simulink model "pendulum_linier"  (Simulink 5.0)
settings: Solver=ode45  StartTime=0.0  StopTime=25  RelTol=1e-6
libraries: simulink x1

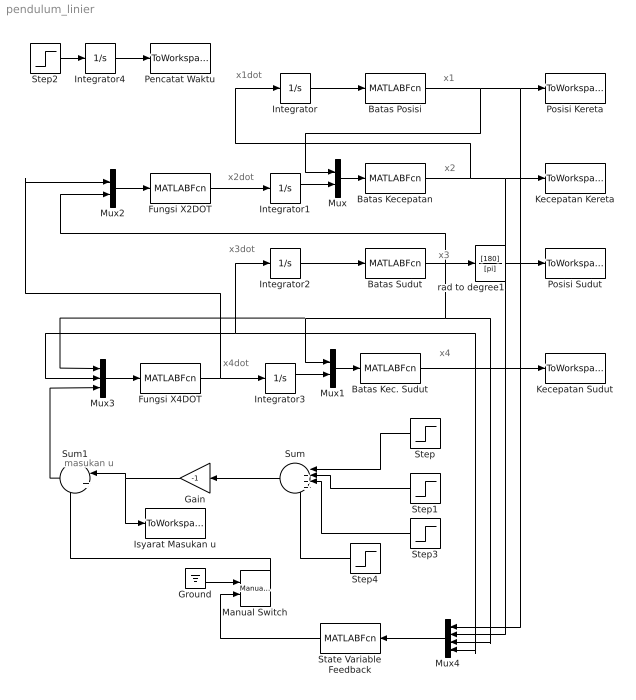
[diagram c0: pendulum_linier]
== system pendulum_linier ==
  note: x1
  note: x2
  note: x3
  note: x4
  note: x1dot
  note: x2dot
  note: x3dot
  note: x4dot
  note: masukan u
  Batas Kec. Sudut : MATLABFcn  MATLABFcn=batas_tetadot
  Batas Kecepatan : MATLABFcn  MATLABFcn=batas_xdot
  Batas Posisi : MATLABFcn  MATLABFcn=batas_x
  Batas Sudut : MATLABFcn  MATLABFcn=batas_teta
  Fungsi X2DOT : MATLABFcn  MATLABFcn=x2dot_lin
  Fungsi X4DOT : MATLABFcn  MATLABFcn=x4dot_lin
  Gain : Gain  Orientation=left  Gain=-1
  Ground : Ground
  Integrator{,1..4} (5 alike) : Integrator
  Isyarat Masukan u : ToWorkspace  VariableName=u  SampleTime=-1  SaveFormat=Array
  Kecepatan Kereta : ToWorkspace  VariableName=kecepatan  SampleTime=-1  SaveFormat=Array
  Kecepatan Sudut : ToWorkspace  VariableName=omega  SampleTime=-1  SaveFormat=Array
  Manual Switch : simulink/Signal Routing/Manual Switch  sw=0  action=0
  Mux : Mux  Inputs=2
  Mux1 : Mux  Inputs=2
  Mux2 : Mux  Inputs=2
  Mux3 : Mux  Inputs=3
  Mux4 : Mux  Orientation=left
  Pencatat Waktu : ToWorkspace  VariableName=time  SampleTime=-1  SaveFormat=Array
  Posisi Kereta : ToWorkspace  VariableName=posisi  SampleTime=-1  SaveFormat=Array
  Posisi Sudut : ToWorkspace  VariableName=teta  SampleTime=-1  SaveFormat=Array
  State Variable Feedback : MATLABFcn  Orientation=left  MATLABFcn=state_control
  Step : Step  Orientation=left  Time=0.1  SampleTime=0
  Step1 : Step  Orientation=left  Time=2  After=-3  SampleTime=0
  Step2 : Step  Time=0  SampleTime=0
  Step3 : Step  Orientation=left  Time=8  After=10  SampleTime=0
  Step4 : Step  Orientation=left  Time=10  After=-8  SampleTime=0  ZeroCross=off
  Sum : Sum  Orientation=left  Inputs=|++++
  Sum1 : Sum  Orientation=left  Inputs=|+-
  rad to degree1 : TransferFcn  Numerator=[180]  Denominator=[pi]
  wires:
  Batas Posisi/1 -> Mux/1, Posisi Kereta/1, Mux4/1
  Batas Kecepatan/1 -> Integrator/1, Kecepatan Kereta/1, Mux4/2
  Batas Sudut/1 -> rad to degree1/1, Mux2/2, Mux1/1, Mux3/1, Mux4/3
  Batas Kec. Sudut/1 -> Kecepatan Sudut/1, Integrator2/1, Mux3/2, Mux4/4
  Integrator/1 -> Batas Posisi/1
  Mux/1 -> Batas Kecepatan/1
  Mux1/1 -> Batas Kec. Sudut/1
  rad to degree1/1 -> Posisi Sudut/1
  Integrator2/1 -> Batas Sudut/1
  Integrator3/1 -> Mux1/2
  Integrator1/1 -> Mux/2
  Fungsi X2DOT/1 -> Integrator1/1
  Fungsi X4DOT/1 -> Integrator3/1, Mux2/1
  Mux2/1 -> Fungsi X2DOT/1
  Mux3/1 -> Fungsi X4DOT/1
  Sum/1 -> Gain/1
  Step/1 -> Sum/1
  Step1/1 -> Sum/2
  Step2/1 -> Integrator4/1
  Integrator4/1 -> Pencatat Waktu/1
  Step3/1 -> Sum/3
  Step4/1 -> Sum/4
  Mux4/1 -> State Variable Feedback/1
  Ground/1 -> Manual Switch/1
  State Variable Feedback/1 -> Manual Switch/2
  Gain/1 -> Isyarat Masukan u/1, Sum1/1
  Sum1/1 -> Mux3/3
  Manual Switch/1 -> Sum1/2
